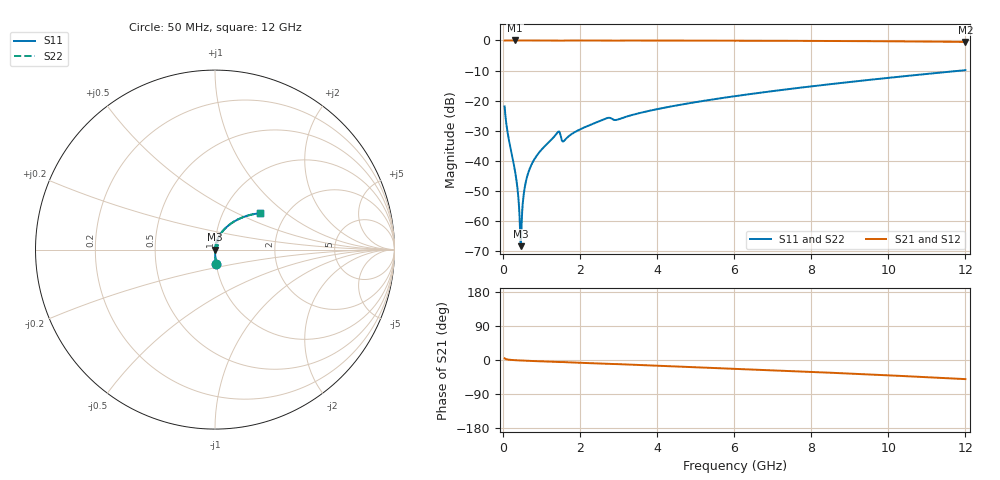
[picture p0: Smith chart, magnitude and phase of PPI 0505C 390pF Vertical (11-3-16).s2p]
# GHz S MA R 50
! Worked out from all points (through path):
!   1601 points, 50 MHz to 12 GHz, reference 50 ohm
!   highest |S21| = 0.00 dB at 318.9 MHz (marker M1); lowest = -0.5 dB at 12 GHz (marker M2)
!   group delay of S21, straight-line fit = 11.6 ps
!   lowest |S11| = -68.3 dB at 468.2 MHz (marker M3), VSWR 1.00, Z = 50 + j0.00419 ohm
!   |S11| at or under -10 dB: start of sweep to 11.9 GHz
!   |S22| runs from -68.3 to -9.9 dB; largest |S21 - S12| = 0
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0.05  0.08034 -85.4  0.9966 4.5  0.9966 4.5  0.08034 -85.4
0.1620312  0.02214 -88.5  0.9995 0.8  0.9995 0.8  0.02214 -88.5
0.318875  0.006845 -87.7  0.9996 -0.5  0.9996 -0.5  0.006845 -87.7
0.3711563  0.004071 -85.8  0.9996 -0.8  0.9996 -0.8  0.004071 -85.8
0.4309062  0.001456 -76.4  0.9996 -1.1  0.9996 -1.1  0.001456 -76.4
0.46825  0.0003836 6.3  0.9996 -1.3  0.9996 -1.3  0.0003836 6.3
0.5055937  0.001454 72.9  0.9996 -1.5  0.9996 -1.5  0.001454 72.9
0.5653438  0.003413 81.4  0.9995 -1.7  0.9995 -1.7  0.003413 81.4
0.6250938  0.005239 83.3  0.9995 -2.0  0.9995 -2.0  0.005239 83.3
0.7296563  0.008193 84.4  0.9995 -2.5  0.9995 -2.5  0.008193 84.4
0.8715625  0.01192 84.5  0.9994 -3.1  0.9994 -3.1  0.01192 84.5
1.416781  0.02944 74.8  0.9945 -5.5  0.9945 -5.5  0.02944 74.8
1.461594  0.03071 65.2  0.9894 -5.6  0.9894 -5.6  0.03071 65.2
1.588563  0.02144 72.0  0.995 -5.5  0.995 -5.5  0.02144 72.0
2.044156  0.03426 80.7  0.9982 -7.5  0.9982 -7.5  0.03426 80.7
2.708875  0.05141 74.1  0.9935 -10.3  0.9935 -10.3  0.05141 74.1
2.962813  0.04809 73.0  0.9934 -10.8  0.9934 -10.8  0.04809 73.0
4.038312  0.07302 73.9  0.9959 -15.1  0.9959 -15.1  0.07302 73.9
6.025  0.1188 66.3  0.9913 -23.1  0.9913 -23.1  0.1188 66.3
8.019156  0.1732 58.1  0.9829 -31.5  0.9829 -31.5  0.1732 58.1
10.01331  0.2398 49.0  0.9685 -40.5  0.9685 -40.5  0.2398 49.0
12  0.3209 39.2  0.9443 -50.5  0.9443 -50.5  0.3209 39.2
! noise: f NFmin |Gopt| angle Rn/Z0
0.05  0.0003104  0.8329  0.2135  0.000392
1.372  0.006027  0.7718  3.679  0.005383
2.701  0.01135  0.763  7.224  0.009687
4.031  0.007259  0.5233  10  0.002653
5.36  0.008483  0.4763  12.76  0.002724
6.682  0.009973  0.4553  15.41  0.003021
8.012  0.01158  0.4451  17.96  0.003399
9.341  0.0133  0.4424  20.43  0.003856
10.67  0.01519  0.446  22.84  0.004411
12  0.01728  0.4552  25.25  0.005096
